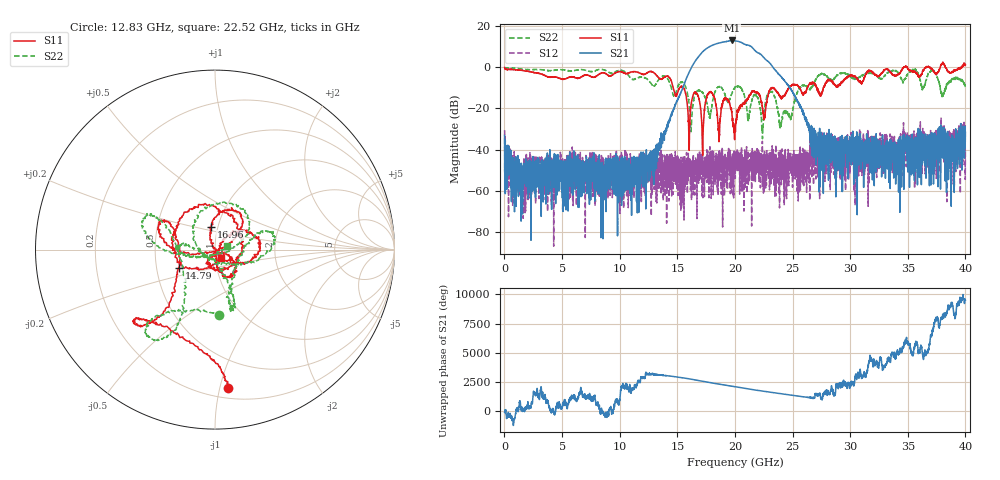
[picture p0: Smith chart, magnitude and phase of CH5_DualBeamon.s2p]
!Keysight Technologies,N5245B,MY57181321,A.14.80.03
!Date: Thursday, March 28, 2024 19:45:44
!Correction: S11(C  2-Port  )
!S21(C  2-Port  )
!S12(C  2-Port  )
!S22(C  2-Port  )
!S2P File: Measurements: S11, S21, S12, S22:
# Hz S  RI  R 50
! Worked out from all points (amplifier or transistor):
!   4000 points, 10 MHz to 40 GHz, reference 50 ohm
!   highest |S21| = 13.0 dB at 19.73 GHz (marker M1)
!   |S21| within 3 dB of that: 17.8 GHz to 21.42 GHz (3.617 GHz wide, 18.4 % of centre)
!   unconditionally stable (mu >= 1): start of sweep to 34.65 GHz; 34.96 GHz to 36.57 GHz; 38.27 GHz to 39.63 GHz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
!   at 6.67 GHz: K = 12718.25, MAG = -42.6 dB, |S12| = -53.9 dB
!   at 20.01 GHz: K = 26.94, MAG = 13.3 dB, |S12| = -48.4 dB
!   at 40 GHz: K = -525.94, MSG = 4.1 dB, |S12| = -39.9 dB
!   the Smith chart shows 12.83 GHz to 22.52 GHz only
!   S11 on the Smith chart (normalised r, x): 12.83 GHz: 0.28, -1.06; 14.79 GHz: 0.65, -0.14; 16.96 GHz: 0.93, +0.24; 22.52 GHz: 1.06, -0.10
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1e7  0.9891 -0.048  -0.00883 -0.0202  -0.0287 0.00751  -0.9266 0.0798
6.68e9  0.2943 0.5063  -0.00398 -0.000473  -0.00438 0.00261  0.8118 0.3355
1.283e10  0.0704 -0.7701  0.00204 -0.00435  0.00345 0.000169  0.0246 -0.3658
1.334e10  -0.067 -0.5702  -0.0093 -0.00389  -0.00432 -0.000371  -0.3036 -0.3708
1.479e10  -0.2011 -0.1009  0.0375 0.1125  0.00219 0.00285  -0.2039 0.00208
1.612e10  0.0686 0.0239  -0.5158 -0.6862  0.000192 0.00582  -0.0408 -0.0307
1.696e10  -0.0216 0.1257  0.2752 1.975  0.00234 0.000675  0.0812 0.2573
1.749e10  0.1431 -0.0705  2.741 -0.5546  0.00525 0.000212  -0.1245 0.1022
1.795e10  0.2397 0.0671  -0.0918 -3.346  -0.00174 -0.00431  0.055 -0.0758
1.854e10  0.0244 0.0224  -3.771 0.6773  -0.000746 0.000196  0.327 0.0446
1.912e10  0.0897 -0.1542  0.875 4.071  -0.00217 0.0066  0.221 0.0625
1.946e10  0.1199 -0.0905  4.06 1.627  -0.00499 -0.00388  0.1196 -0.085
1.973e10  0.0785 -0.0297  4.15 -1.714  -0.00402 0.00153  0.0895 -0.2053
2.001e10  -0.0111 -0.0359  1.602 -4.079  0.00341 0.00165  0.0926 -0.3111
2.061e10  0.0556 -0.1061  -3.766 -1.122  -0.00428 0.000118  0.1011 -0.2601
2.12e10  0.1037 0.1545  -0.5781 3.366  0.00283 6.49e-06  -0.0456 -0.0337
2.177e10  -0.2161 0.1294  2.44 0.5576  0.00155 5.1e-05  -0.2136 0.0148
2.252e10  0.0333 -0.0457  -0.2192 -1.69  0.00423 -0.0061  0.0695 0.0212
2.355e10  -0.1599 0.227  -0.3612 0.7454  0.0104 -0.00757  0.00268 0.1509
2.667e10  0.1441 0.3729  0.00331 0.00636  -0.00213 -0.00053  0.05 0.3195
3.334e10  0.4512 0.7327  -0.0112 0.0101  0.0104 -0.01  0.7439 -0.1983
4e10  0.9464 0.6493  -0.0204 0.0166  0.00202 0.00996  0.0363 -0.3333
